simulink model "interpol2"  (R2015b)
settings: Solver=VariableStepAuto  StartTime=0.0  StopTime=10.0  RelTol=1e-3
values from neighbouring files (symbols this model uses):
  a = 1/(Tsig/2.5)    (= 7.8125)    [fourier_transf_puls_3.m]    (also in fourier_transf_puls_4.m; schar_1.m = 5)
  b = 10    [schar_1.m]
  hint = fir1(nord, 0.9*1/L)    [interpol_1.m]    (also in interpol_2.m = fir1(nord, 1/L); poly_interp_1.m = fir1(nord2, 1/L); poly_interp_2.m = fir1(nord2, 1/L))
  L = 3    [farrow_3.m]    (also in farrow_4.m = 480; ifir_1.m = 5; ifir_dezim_1.m = 5; ifir_high1.m = 5)
  nord = 6    [dezimier_1.m]    (also in dezimier_11.m; dezimier_2.m = 256; dezimier_3.m = 256; farrow_2.m = 128)
  Ts = 1/fs    (= 5e-05)    [basisband_1.m]    (also in basisband_2.m = 5e-06; dezimier_1.m = 0.0005; dezimier_11.m = 0.0005; dezimier_2.m = 0.0005)
libraries: dspsigops x2

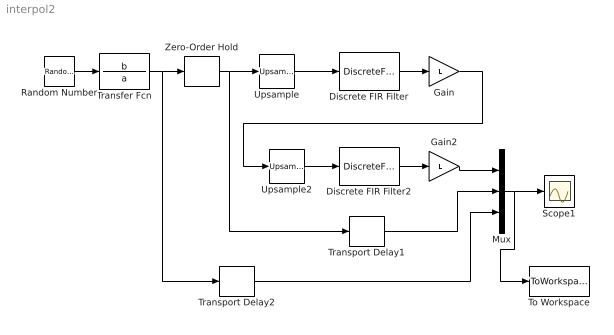
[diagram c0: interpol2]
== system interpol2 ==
  Discrete FIR Filter : DiscreteFir  Coefficients=hint
  Discrete FIR Filter2 : DiscreteFir  Coefficients=hint
  Gain : Gain  Gain=L
  Gain2 : Gain  Gain=L
  Mux : Mux  Inputs=3
  Random Number : RandomNumber  Seed=03678  SampleTime=0
  Scope1 : Scope
  To Workspace : ToWorkspace  VariableName=y  SaveFormat=Timeseries  SampleTime=-1
  Transfer Fcn : TransferFcn  Numerator=b  Denominator=a
  Transport Delay1 : TransportDelay  DelayTime=(nord/2)*(Ts/L)*(1+1/L)  BufferSize=1024*4
  Transport Delay2 : TransportDelay  DelayTime=(nord/2)*(Ts/L)*(1+1/L)  BufferSize=1024*4
  Upsample : dspsigops/Upsample  N=L  phase=0  RateOptions=Allow multirate processing  ic=0  mode=Unused parameter value
  Upsample2 : dspsigops/Upsample  N=L  phase=0  RateOptions=Allow multirate processing  ic=0  mode=Unused parameter value
  Zero-Order Hold : ZeroOrderHold  SampleTime=Ts
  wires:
  Random Number/1 -> Transfer Fcn/1
  Upsample/1 -> Discrete FIR Filter/1
  Discrete FIR Filter/1 -> Gain/1
  Transfer Fcn/1 -> Transport Delay2/1, Zero-Order Hold/1
  Mux/1 -> To Workspace/1, Scope1/1
  Zero-Order Hold/1 -> Transport Delay1/1, Upsample/1
  Upsample2/1 -> Discrete FIR Filter2/1
  Discrete FIR Filter2/1 -> Gain2/1
  Gain/1 -> Upsample2/1
  Gain2/1 -> Mux/1
  Transport Delay2/1 -> Mux/3
  Transport Delay1/1 -> Mux/2
